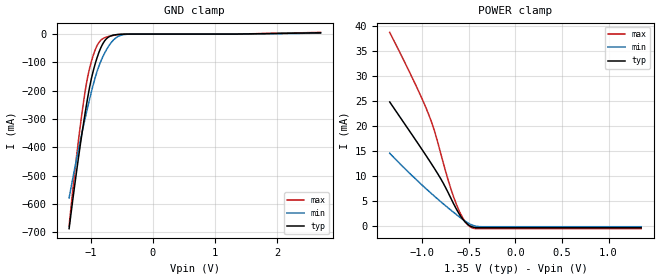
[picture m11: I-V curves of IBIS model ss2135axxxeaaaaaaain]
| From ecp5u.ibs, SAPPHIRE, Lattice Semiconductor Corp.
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|   Model ss2135axxxeaaaaaaain
[Model] ss2135axxxeaaaaaaain
Model_type Input
Polarity   Non-Inverting
Vinl =  0.575V
Vinh =  0.775V
C_comp   3.896pF   3.894pF   3.903pF
[Temperature Range]   25.000   0.125k   -40.000
[Voltage Range]   1.350V   1.280V   1.420V
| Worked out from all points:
|   GND clamp passes 1 mA (typ) near -0.54 V on its own axis
|   POWER clamp passes 1 mA (typ) near -0.55 V on its own axis
[GND_clamp]
|Voltage   I(typ)   I(min)   I(max)
-1.35V    -687.3mA   -578.9mA   -678.2mA
-1.26V    -534.4mA   -475.1mA   -489.7mA
-1.2V     -438.1mA   -409.1mA   -376.7mA
-1.08V    -262.9mA   -286.2mA   -186mA
-1.02V    -187.7mA   -230mA     -120.8mA
-960mV    -129.1mA   -177.6mA   -74.01mA
-900mV    -83.64mA   -132.1mA   -40.81mA
-810mV    -35.24mA   -81.59mA   -16.5mA
-720mV    -11.12mA   -44.72mA   -8.737mA
-630mV    -3.4mA     -19.67mA   -4.118mA
-450mV    -169.7uA   -1.25mA    -168.1uA
2.7V      4.573mA    3.195mA    5.981mA
[POWER_clamp]
|Voltage   I(typ)   I(min)   I(max)
-1.35V    24.83mA    14.55mA    38.8mA
-1.08V    17.43mA    9.524mA    28.6mA
-930mV    13.23mA    6.926mA    22.26mA
-870mV    11.5mA     5.927mA    19.05mA
-750mV    7.661mA    4.003mA    10.92mA
-660mV    4.26mA     2.628mA    5.576mA
-600mV    2.242mA    1.748mA    2.805mA
-570mV    1.419mA    1.323mA    1.7mA
-510mV    230.3uA    557.6uA    138.8uA
-450mV    -318.8uA   33.91uA    -516.7uA
-360mV    -408uA     -196.9uA   -584.4uA
1.35V     -408uA     -196.9uA   -584.4uA
